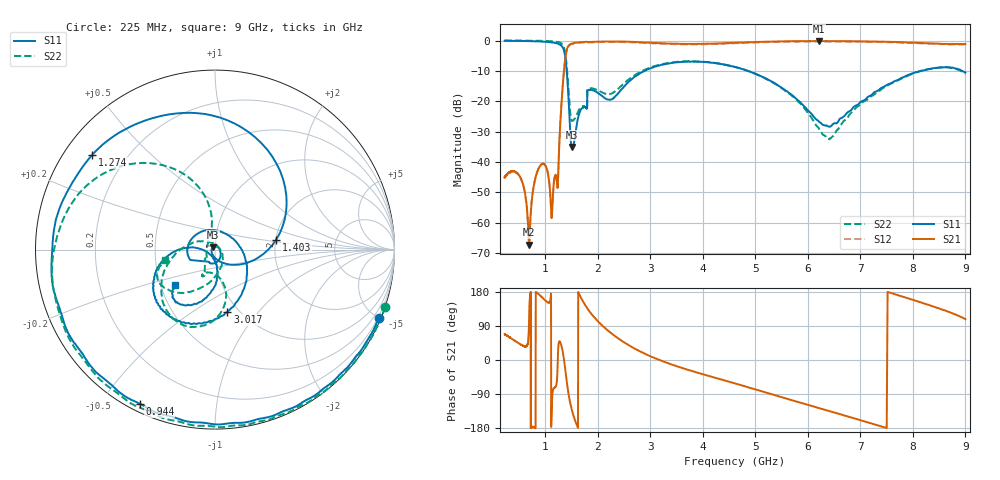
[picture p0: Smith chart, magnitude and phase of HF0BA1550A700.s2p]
!Agilent Technologies,E8358A,US41080443,A.07.50.56
!Agilent E8358A: A.07.50.56
!Date: Wednesday, May 04, 2016 15:11:22
!Correction: S11(Full 2 Port(1,2))
!S21(Full 2 Port(1,2))
!S12(Full 2 Port(1,2))
!S22(Full 2 Port(1,2))
!S2P File: Measurements: S11, S21, S12, S22:Log Frequency Sweep
# Hz S  dB  R 50
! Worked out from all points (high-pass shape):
!   1601 points, 225 MHz to 9 GHz, reference 50 ohm
!   highest |S21| = -0.17 dB at 6.209 GHz (marker M1); lowest = -67.2 dB at 689.9 MHz (marker M2)
!   |S21| within 3 dB of the highest: 1.408 GHz to end of sweep
!   lowest |S11| = -35.1 dB at 1.507 GHz (marker M3), VSWR 1.04, Z = 48.8 + j1.24 ohm
!   |S11| at or under -10 dB: 1.407 GHz to 2.892 GHz (1.484 GHz wide, 69.1 % of centre); 4.858 GHz to 8.156 GHz (3.298 GHz wide, 50.7 % of centre); 8.937 GHz to end of sweep
!   |S22| runs from -32.6 to 0.0 dB; largest |S21 - S12| = 0.021
!   S11 on the Smith chart (normalised r, x): 225 MHz: 0.13, -4.99; 944 MHz: 0.03, -0.62; 1.274 GHz: 0.08, +0.34; 1.403 GHz: 2.01, +0.25; 3.017 GHz: 0.89, -0.70; 9 GHz: 0.60, -0.26
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2.25e8  -0.09 -22.6  -45.10 68.3  -45.30 68.7  0.02 -18.8
5.428431e8  -0.15 -57.4  -45.71 39.8  -45.95 40.0  -0.02 -46.9
6.306059e8  -0.20 -68.1  -52.16 35.8  -52.29 36.3  -0.06 -55.3
6.899351e8  -0.23 -75.9  -67.22 103.6  -67.53 102.1  -0.07 -61.5
7.814078e8  -0.23 -88.9  -47.75 -177.5  -47.89 -176.8  -0.06 -71.6
9.440247e8  -0.39 -116.1  -40.59 164.7  -40.74 164.6  -0.15 -92.4
1.044816e9  -0.46 -137.4  -43.31 151.6  -43.44 152.0  -0.16 -108.1
1.122225e9  -0.65 -157.2  -58.14 -132.0  -58.40 -134.0  -0.27 -122.6
1.233482e9  -0.99 162.9  -48.54 -17.9  -48.64 -17.6  -0.45 -150.5
1.273945e9  -1.27 142.4  -31.02 49.3  -31.20 49.6  -0.64 -164.6
1.340229e9  -2.54 91.1  -12.94 15.4  -13.11 15.7  -1.61 160.2
1.403475e9  -9.24 9.2  -3.46 -51.6  -3.61 -51.4  -7.59 109.2
1.507456e9  -35.05 133.9  -1.01 -132.7  -1.16 -132.6  -26.48 162.9
1.687749e9  -22.47 -89.6  -0.53 162.1  -0.69 162.3  -21.82 -130.2
2.12538e9  -18.88 105.7  -0.33 85.8  -0.48 85.9  -17.40 -109.1
3.017395e9  -9.04 -78.7  -0.73 8.9  -0.90 9.0  -8.75 -86.5
3.152512e9  -8.28 -88.8  -0.85 1.1  -1.01 1.2  -8.05 -91.3
4.622431e9  -8.76 -156.8  -0.76 -62.1  -0.91 -62.0  -8.73 -145.2
6.081681e9  -24.41 -175.5  -0.18 -121.6  -0.35 -121.7  -25.78 126.2
6.209194e9  -26.70 -162.2  -0.17 -126.8  -0.34 -126.8  -28.90 102.1
7.553438e9  -14.29 -88.9  -0.44 178.0  -0.60 178.2  -14.43 -100.5
9e9  -10.54 -138.1  -1.15 108.0  -1.29 108.3  -10.98 -167.6
